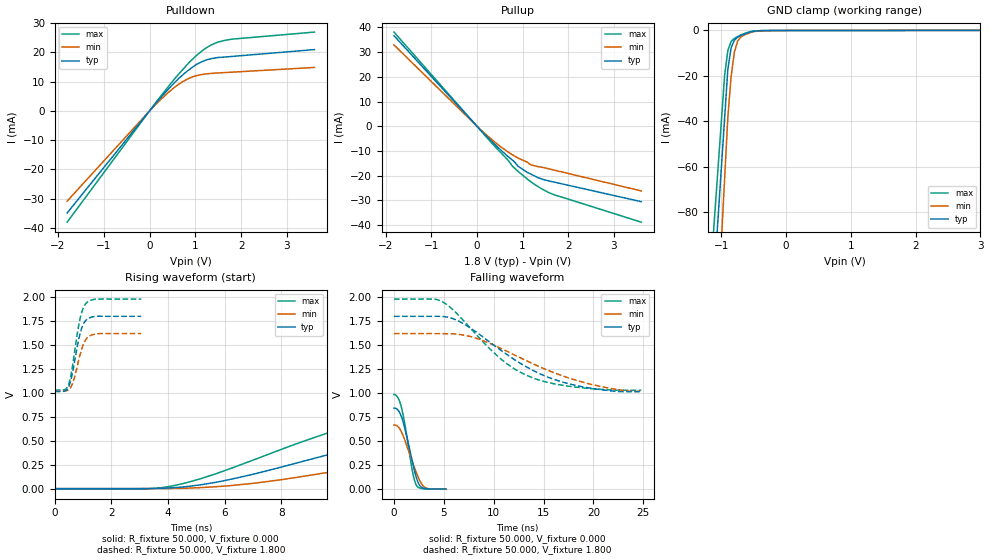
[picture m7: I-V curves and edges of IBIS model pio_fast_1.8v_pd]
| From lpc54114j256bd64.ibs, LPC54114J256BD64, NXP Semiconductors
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[Model]   pio_fast_1.8v_pd
Model_type I/O
Vinl=4.000E-01
Vinh=1.500E+00
Vref=0.000E+00
Rref=1.000E+06
Cref=2.000E-11
Vmeas=9.000E-01
C_comp   9.060E-12   8.700E-12   9.420E-12
[Voltage Range]   1.800E+00   1.620E+00   1.980E+00
[POWER Clamp Reference]   1.800E+00   1.620E+00   1.980E+00
[GND Clamp Reference]   0.000E+00   0.000E+00   0.000E+00
[Pullup Reference]   1.800E+00   1.620E+00   1.980E+00
[Pulldown Reference]   0.000E+00   0.000E+00   0.000E+00
[Temperature Range]   25   105   -40
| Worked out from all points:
|   slope of the pulldown table from 0 to 0.27 V, typ, clamps not added: 54.4 ohm
|   slope of the pullup table from 0 to 0.27 V, typ, clamps not added: 52.3 ohm
|   GND clamp passes 1 mA (typ) near -0.59 V on its own axis
|   rising waveform, R_fixture 50.000, V_fixture 0.000: 20-80 % time 7.6ns typ, 8.94ns min, 6.14ns max; typ from 0 V to 0.844 V
|   falling waveform, R_fixture 50.000, V_fixture 0.000: 20-80 % time 1.13ns typ, 1.38ns min, 947ps max; typ from 0.844 V to 0 V
|   rising waveform, R_fixture 50.000, V_fixture 1.800: 20-80 % time 315ps typ, 326ps min, 312ps max; typ from 1.01 V to 1.8 V
|   falling waveform, R_fixture 50.000, V_fixture 1.800: 20-80 % time 7.15ns typ, 8.09ns min, 5.95ns max; typ from 1.8 V to 1.01 V
[GND Clamp]
-1.8V     -407.8mA   -530.1mA   -362mA
-950mV    -38.84mA   -65.54mA   -19.87mA
-900mV    -17.14mA   -38.22mA   -8.822mA
-850mV    -7.714mA   -20.45mA   -4.848mA
-800mV    -4.295mA   -9.707mA   -3.501mA
-750mV    -2.992mA   -4.775mA   -2.724mA
-700mV    -2.198mA   -2.883mA   -1.947mA
-550mV    -629.8uA   -893.1uA   -475.4uA
-450mV    -202.6uA   -255.3uA   -151.7uA
3.6V      64.79uA    77.25uA    67.44uA
[Power Clamp]
-1.8V     0A         0A         0A
0V        0A         0A         0A
1.8V      0A         0A         0A
3.6V      0A         0A         0A
[Pullup]
-1.82V    36.68mA    32.95mA    38.14mA
60mV      -1.186mA   -1.045mA   -1.256mA
520mV     -9.605mA   -8.289mA   -10.63mA
680mV     -12.23mA   -10.39mA   -13.75mA
780mV     -13.74mA   -11.58mA   -16.2mA
900mV     -16.13mA   -12.84mA   -18.25mA
1V        -17.45mA   -13.7mA    -19.78mA
1.2V      -19.53mA   -15.73mA   -22.73mA
1.42V     -21.36mA   -16.58mA   -25.34mA
1.62V     -22.32mA   -17.43mA   -27.21mA
3.6V      -30.52mA   -26.17mA   -38.83mA
[Pulldown]
-1.8V     -34.9mA    -30.86mA   -38.06mA
0V        0A         0A         0A
400mV     7.25mA     6.14mA     8.117mA
600mV     10.52mA    8.704mA    11.94mA
820mV     13.55mA    10.8mA     15.78mA
1.02V     15.83mA    12.03mA    18.86mA
1.16V     16.92mA    12.47mA    20.67mA
1.32V     17.75mA    12.77mA    22.31mA
1.48V     18.2mA     12.94mA    23.43mA
1.8V      18.6mA     13.23mA    24.51mA
3.6V      20.95mA    14.84mA    26.92mA
[Rising Waveform]
R_fixture = 50.000
V_fixture = 0.000
V_fixture_min = 0.000
V_fixture_max = 0.000
|  time   V(typ)   V(min)   V(max)
0s        34.77uV    885.7uV    -5.148mV
3.15ns    1.061mV    1.133mV    -3.175mV
4.25ns    11.2mV     2.73mV     34.99mV
6.25ns    100.2mV    33.35mV    215.6mV
10.3ns    404.7mV    203mV      644.2mV
11.85ns   514.3mV    282.8mV    763.1mV
13.5ns    612.1mV    364.3mV    849.4mV
16ns      718mV      470.9mV    919.6mV
18.35ns   777mV      549.1mV    952.7mV
25.05ns   843.5mV    666.2mV    979.7mV
[Falling Waveform]
R_fixture = 50.000
V_fixture = 0.000
V_fixture_min = 0.000
V_fixture_max = 0.000
|  time   V(typ)   V(min)   V(max)
0s        843.5mV    666.2mV    984.7mV
400ps     824mV      651.7mV    951mV
750ps     753.1mV    595.5mV    851.3mV
1.15ns    604.7mV    492.1mV    641.1mV
1.85ns    283.2mV    284.8mV    189mV
2.05ns    194mV      225.8mV    95mV
2.25ns    117.7mV    169.1mV    39.54mV
2.6ns     34.93mV    85.04mV    9.538mV
3.15ns    5.305mV    14.58mV    -614.4uV
5.2ns     34.77uV    885.7uV    147.6uV
[Rising Waveform]
R_fixture = 50.000
V_fixture = 1.800
V_fixture_min = 1.620
V_fixture_max = 1.980
|  time   V(typ)   V(min)   V(max)
0s        1.014V     1.019V     1.03V
350ps     1.019V     1.02V      1.035V
500ps     1.069V     1.035V     1.099V
650ps     1.246V     1.116V     1.327V
800ps     1.495V     1.287V     1.629V
900ps     1.628V     1.408V     1.785V
1ns       1.714V     1.501V     1.884V
1.1ns     1.759V     1.559V     1.935V
1.55ns    1.801V     1.619V     1.98V
3.05ns    1.8V       1.62V      1.98V
[Falling Waveform]
R_fixture = 50.000
V_fixture = 1.800
V_fixture_min = 1.620
V_fixture_max = 1.980
|  time   V(typ)   V(min)   V(max)
0s        1.8V       1.62V      1.98V
4ns       1.8V       1.62V      1.98V
4.95ns    1.798V     1.619V     1.946V
7.05ns    1.718V     1.603V     1.747V
10.75ns   1.444V     1.464V     1.354V
12.2ns    1.341V     1.391V     1.244V
13.95ns   1.236V     1.305V     1.157V
18.75ns   1.069V     1.119V     1.056V
22.65ns   1.015V     1.032V     1.03V
24.8ns    1.014V     1.019V     1.03V
[Ramp]
dV/dt_r   5.0453E-01/7.5936E-09   4.0062E-01/8.9309E-09   5.9090E-01/6.1396E-09
dV/dt_f   4.7142E-01/7.1409E-09   3.6076E-01/8.0730E-09   5.6989E-01/5.9432E-09
R_load = 50
